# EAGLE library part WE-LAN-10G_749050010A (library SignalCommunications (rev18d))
WE-LAN 10G Transformer 10Gbit Base-T - Compliant with standards: IEEE 802.3an and upcoming IEEE 802.3bt - SMD -- Ethernet -- Ethernet speed up to 10Gbit/s --Power over Ethernet PoE and PoE+ --10Gbit with ETR and PoE up to 150 W (for industrial applications) Details see: http://katalog.we-online.de/en/pbs/WE-LAN-10G Updated by Dan Xu 2014-07-08 2014 (C) Würth Elektronik
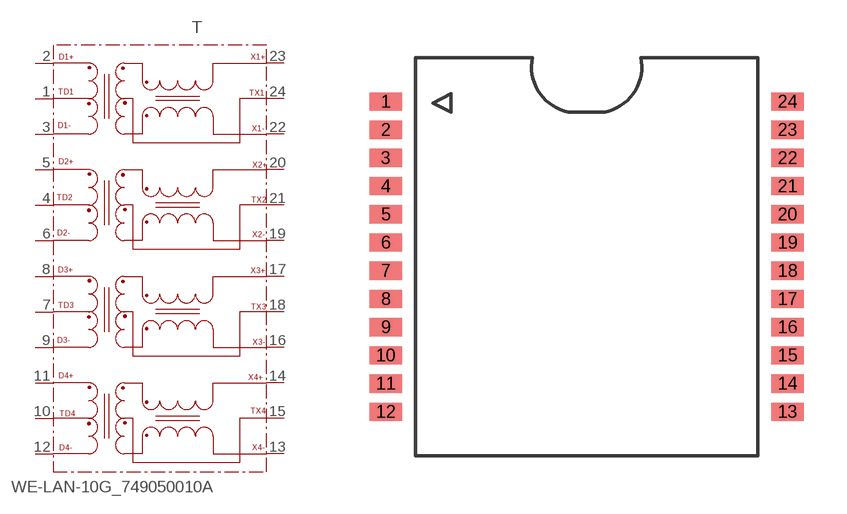
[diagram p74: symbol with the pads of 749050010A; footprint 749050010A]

Designator prefix T

## WE-LAN-10G_749050010A  [749050010A]
1  TD1
2  D1+
3  D1-
4  TD2
5  D2+
6  D2-
7  TD3
8  D3+
9  D3-
10  TD4
11  D4+
12  D4-
13  X4-
14  X4+
15  TX4
16  X3-
17  X3+
18  TX3
19  X2-
20  X2+
21  TX2
22  X1-
23  X1+
24  TX1

## Footprint 749050010A (pad centres in mm)
MAX Height = 6.32 mm
smd 1.14 x 0.64: 1 -7.05,5.445; 2 -7.05,4.455; 3 -7.05,3.465; 4 -7.05,2.475; 5 -7.05,1.485; 6 -7.05,0.495; 7 -7.05,-0.495; 8 -7.05,-1.485; 9 -7.05,-2.475; 10 -7.05,-3.465; 11 -7.05,-4.455; 12 -7.05,-5.445; 13 7.05,-5.445; 14 7.05,-4.455; 15 7.05,-3.465; 16 7.05,-2.475; 17 7.05,-1.485; 18 7.05,-0.495; 19 7.05,0.495; 20 7.05,1.485; 21 7.05,2.475; 22 7.05,3.465; 23 7.05,4.455; 24 7.05,5.445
